(* Logix 5000 AddOnInstructionDefinition export T2DRIVE; software revision 32.02 *)

TYPE Exlar_Control :   // Tritex II Control
STRUCT
   EnableOutputs : INT;   // EnableOutputs
   InputEventsMode : INT;   // 4316
   InputEventsModeLevel : INT;   // 4318
   InputEventsMotion : INT;   // 4317
   HostCommandControlMode : INT;   // 4303
   HostPosition_low : INT;   // 4304
   HostPosition_high : INT;
   HostVelocity_low : INT;   // 4306
   HostVelocity_high : INT;
   HostAcceleration_low : INT;   // 4308
   HostAcceleration_high : INT;
   HostCurrent : INT;   // 4310
   InputEventsMoveEdge : INT;   // 4319
   JogSlowVelocity_low : INT;   // 6022
   JogSlowVelocity_high : INT;
   JogAcceleration_low : INT;   // 6026
   JogAcceleration_high : INT;
   MoveOption : INT;   // 6100
   MoveCurrentLimit : INT;   // 6101
   MoveAcceleration_low : INT;   // 6102
   MoveAcceleration_high : INT;
   MoveDeceleration_low : INT;   // 6500
   MoveDeceleration_high : INT;
   MovePrimaryOption : INT;   // 6106
   spare : INT;   // spare
   MovePrimaryPosition_low : INT;   // 6108
   MovePrimaryPosition_high : INT;
   MovePrimaryVelocity_low : INT;   // 6110
   MovePrimaryVelocity_high : INT;
   MoveSecondaryOption : INT;   // 6112
   spare2 : INT;   // spare
   MoveSecondaryPosition_low : INT;   // 6114
   MoveSecondaryPosition_high : INT;
   MoveSecondaryVelocity_low : INT;   // 6116
   MoveSecondaryVelocity_high : INT;
END_STRUCT
END_TYPE

TYPE Exlar_Drive :   // Tritex II Data
STRUCT
   Control : Exlar_Control;   // Control bits to send to the drive
   Status : Exlar_Status;   // Status bits received from the drive
END_STRUCT
END_TYPE

TYPE Exlar_Status :   // Tritex II Status
STRUCT
   EIP_Comm : INT;   // EIP module communication
   OutputEventsStatus : INT;   // 104
   OutputEventsMoveInPosition : INT;   // 108
   OutputEventsMotion : INT;   // 105
   OutputsEventsMotionActive : INT;   // 107
   PositionFeedback_low : INT;   // 378
   PositionFeedback_high : INT;
   SoftFaults : INT;   // 7
   HardFaults : INT;   // 6
   VelocityDisplay_low : INT;   // 356
   VelocityDisplay_high : INT;
   CurrentDisplay : INT;   // 567
   CurrentContinuous : INT;   // 565
   CurrentLimit : INT;   // 5108
   VoltageHallBattery : INT;   // 8
   VoltageBus : INT;   // 571
   TemperatureBoard : INT;   // 11
   TemperatureActuator : INT;   // 15
END_STRUCT
END_TYPE

ADD_ON_INSTRUCTION T2DRIVE   (* revision 1.0 *)
// Drive Communication
VAR_IN_OUT
   Drive_Input : INT[101]; {required}
   Drive_Output : INT[101]; {required}
   Drive : Exlar_Drive; {required}
END_VAR
VAR_OUTPUT
   ER : BOOL; {access Read Only, visible}   // Fault
   Status : DINT; {access Read Only, visible}   // EIP interface Status
END_VAR
VAR_INPUT
   OutputEnable : BOOL; {access Read Only, visible}
END_VAR

ROUTINE Logic   (* structured text *)
   (***********************************************)
   (*   Exlar Tritex 2 Drive                      *)
   (*                                             *)
   (***********************************************)
   
   	(* Enable EtherNet/IP communication board *)
   	if OutputEnable then
   		Drive.Control.EnableOutputs.0 := 1;
   	else
   		Drive.Control.EnableOutputs.0 := 0;
   	end_if;
   
   
   	(* Note: If Tritex II translation tables length are changed,
   	   CPS data size and data Type needs to change *)
   
   	(* Copy Implicit Input data to PLC Internal register - Default 18 words*)
   	cps(Drive_Input[0],Drive.Status,18);
   
   
   	(* Copy Internal registers to PLC Implicit Output - Default 36 words *)
   	cps(Drive.Control, Drive_Output[0],36);
   
   
   	(* Tritex communication status *)
   	if 	Drive.Status.EIP_Comm.0 or
   		Drive.Status.EIP_Comm.1 or
   		Drive.Status.EIP_Comm.2 then
   		ER := 1;
   	else
   		ER := 0;
   	end_if;
   
   
   	(* Copy  Communication Status registers *)
   		Status := Drive.Status.EIP_Comm;
   		Status := Status AND 16#0000FFFF;
   
   	 (* StatusRegister
   		  	Bit				Description
   			=======			===============================
   			.0				Error - Tritex responded with error code
   							Read Extended Module Status(Object 64h,Instance 1,Attribute 101) for Modbus error
   			.1				Error - Communication between EIP module and Tritex timed-out
   			.2				Error - Communication between EIP module and Tritex cannot be established
   			.3-7			Reserved
   			.8				EIP interface is currently active at factory defaults
   			.9				EIP interface has a new configuration
   			.10-15			Reserved
   	 *)
END_ROUTINE
END_ADD_ON_INSTRUCTION
